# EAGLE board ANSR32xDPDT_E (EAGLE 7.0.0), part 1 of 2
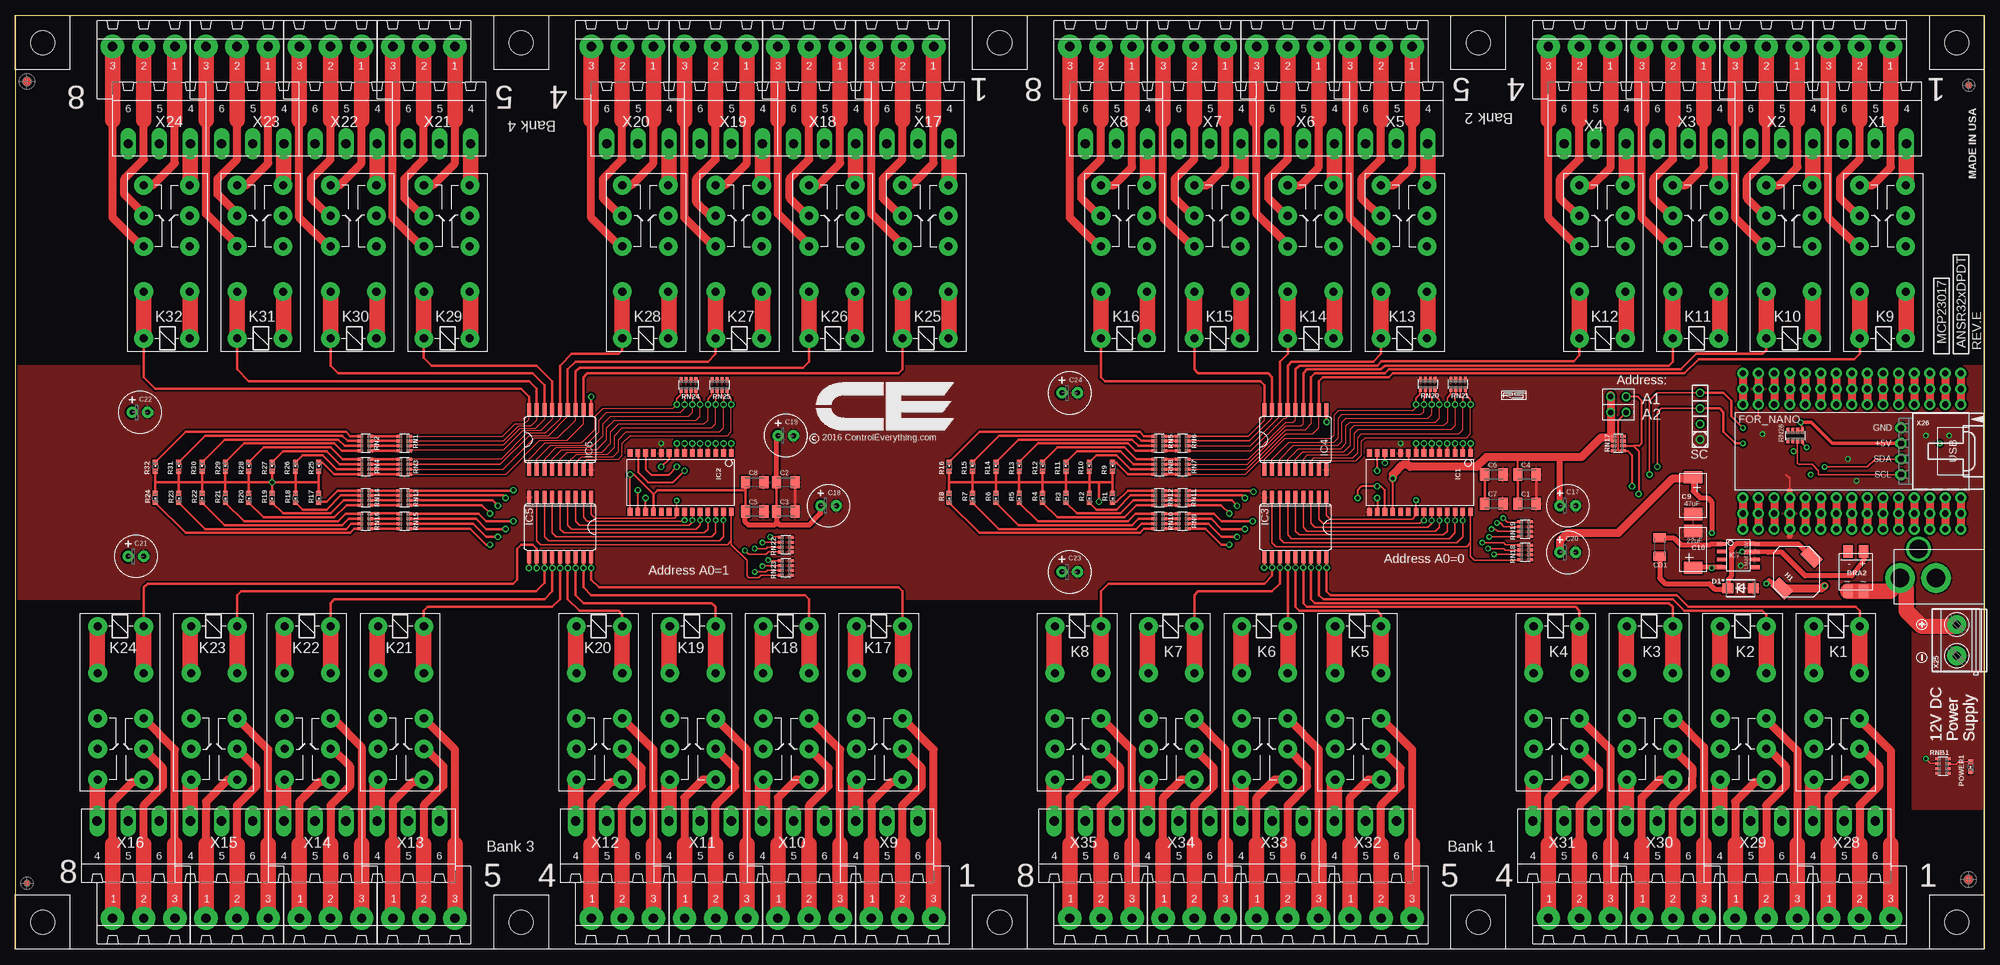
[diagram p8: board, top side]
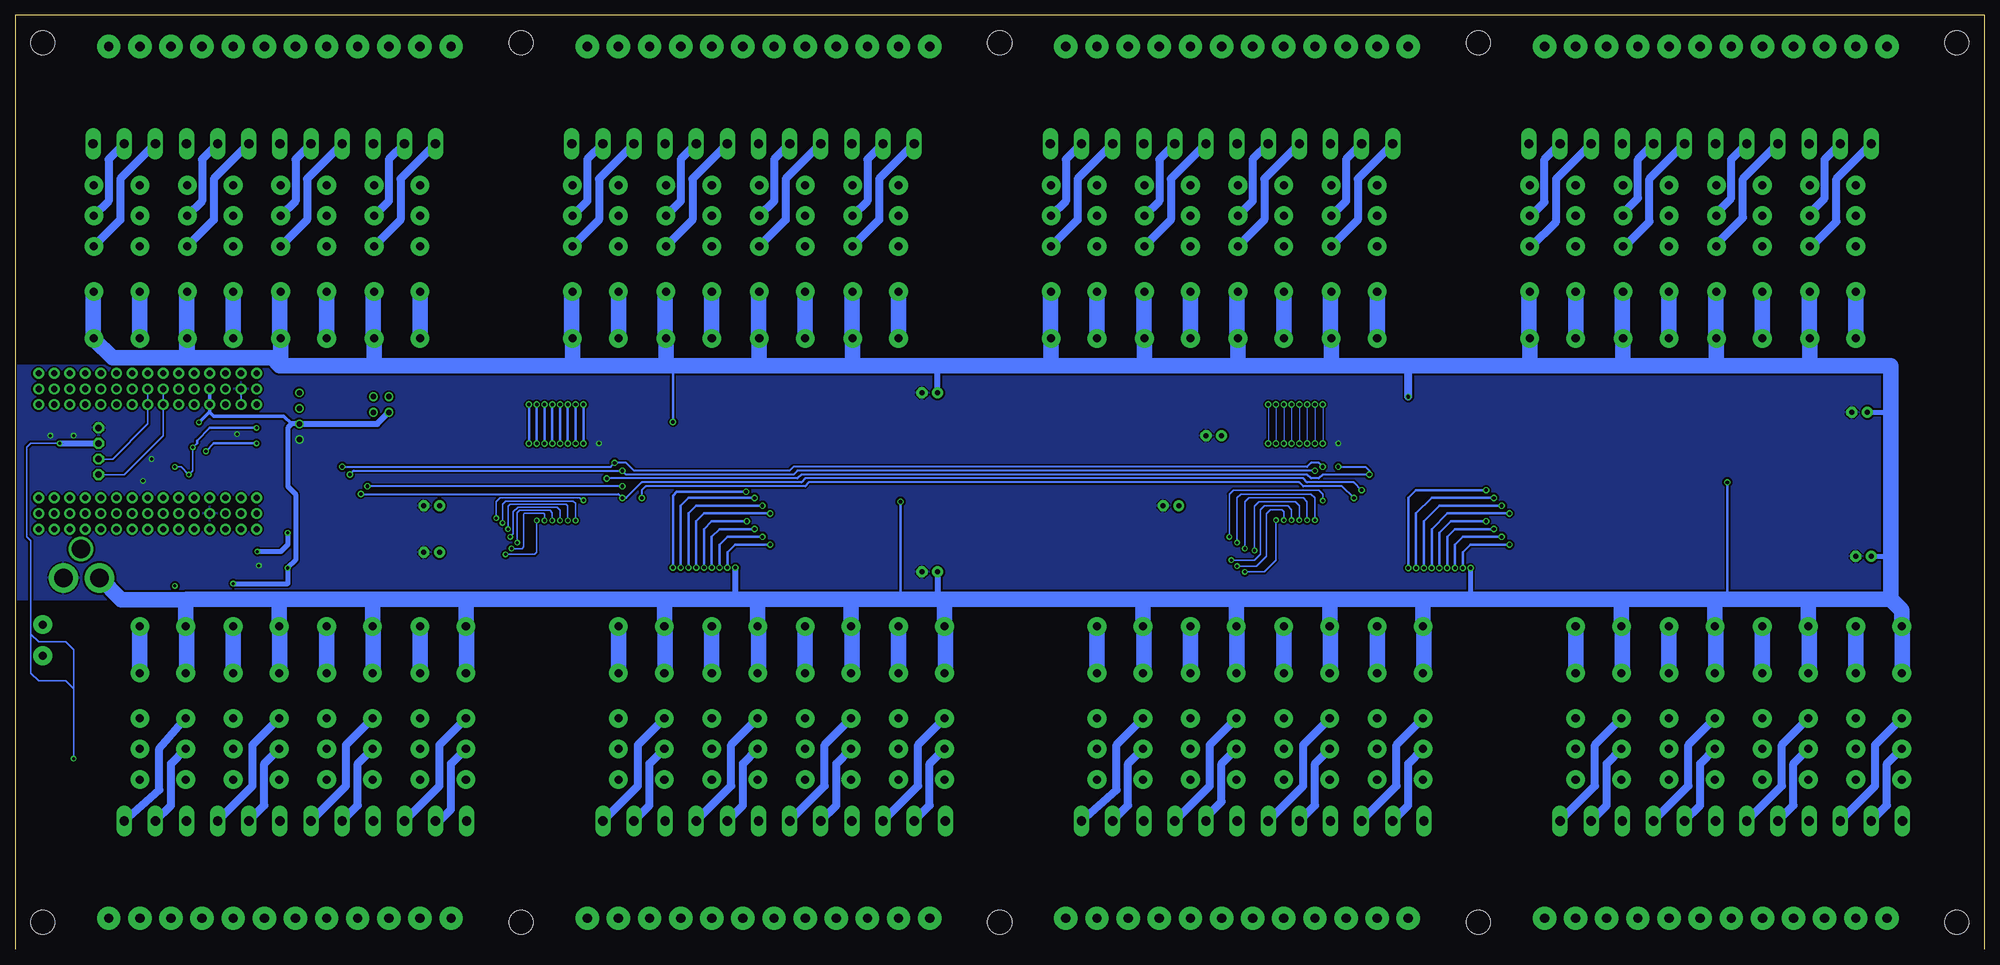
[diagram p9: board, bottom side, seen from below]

Size 321.31 x 152.41 mm. Coordinates in mm from the lower left corner, seen from the top.
Outline: 321.29,0 321.29,152.41 0,152.41 0,0.01
Outline: 321.29,93.99 321.29,13.97
Outline: 321.29,95.26 321.29,14.6
Outline: 321.31,95.26 321.31,37.48
Copper layers (1*16): Top 0.035mm / dielectric 1.5mm / Bottom 0.035mm
Design rules "default": minimum track width 5mil, minimum drill 24mil, track to track 5mil, track to pad 5mil, pad to pad 5mil, via to via 5mil, smd to smd 5mil, copper to edge 10mil, drill to drill 8mil, minimum pad ring 10mil, minimum via ring 8mil, stop-mask expansion 2mil, vias tented up to drill 0mil, thermal gap 10mil

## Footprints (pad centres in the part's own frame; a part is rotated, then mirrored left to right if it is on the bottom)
MB2S = smd 1.55 x 2.1: + 0,-6.5; - 2.54,-6.5; ~@1 0,0; ~@2 2.54,0
_CA_.1UF_50V = smd 1.5 x 2: 1 -1.5,0; 2 1.5,0
_CB_10UF_25V = smd 1.5 x 2: 1 -1.5,0; 2 1.5,0
C2917(7343)-Y = smd 2 x 3: 1 -3,0; 2 3,0
E-025X060 = drill 0.813 pad 1.778: + -1.27,0 | drill 0.813 pad 1.778 octagon: - 1.27,0
_CD_10NF_50V = smd 1.5 x 2: 1 -1.5,0; 2 1.5,0
DO214AC_ZENER = smd 1.8 x 1.7: A 2.05,0; C -2.05,0
ARDUINO_NANO = drill 1 pad 1.778: 3V1 -2.54,-2.54; 3V3 0,-2.54; 5V 0,-27.94; 5V1 -2.54,-27.94; A0 0,-7.62; A1 0,-10.16; A2 0,-12.7; A3 0,-15.24; A4 0,-17.78; A5 0,-20.32; A6 0,-22.86; A7 0,-25.4; A8 -2.54,-7.62; A9 -2.54,-10.16; A10 -2.54,-12.7; A11 -2.54,-15.24; A12 -2.54,-17.78; A13 -2.54,-20.32; A14 -2.54,-22.86; A15 -2.54,-25.4; D1 -2.54,0; D2 20.32,-25.4; D3 20.32,-22.86; D4 20.32,-20.32; D5 20.32,-17.78; D6 20.32,-15.24; D7 20.32,-12.7; D8 20.32,-10.16; D9 20.32,-7.62; D10 20.32,-5.08; D11 20.32,-2.54; D12 20.32,0; D13 0,0; D14 22.86,0; D15 22.86,-2.54; D16 22.86,-5.08; D17 22.86,-7.62; D18 22.86,-10.16; D19 22.86,-12.7; D20 22.86,-15.24; D21 22.86,-17.78; D22 22.86,-20.32; D23 22.86,-22.86; D24 22.86,-25.4; GND 0,-33.02; GND1 -2.54,-33.02; GND@1 20.32,-27.94; GND@2 22.86,-27.94; P$16 2.54,0; P$17 2.54,-2.54; P$18 2.54,-5.08; P$19 2.54,-7.62; P$20 2.54,-10.16; P$21 2.54,-12.7; P$22 2.54,-15.24; P$23 2.54,-17.78; P$24 2.54,-20.32; P$25 2.54,-22.86; P$26 2.54,-25.4; P$27 2.54,-27.94; P$28 2.54,-30.48; P$29 2.54,-33.02; P$30 2.54,-35.56; P$31 17.78,0; P$32 17.78,-2.54; P$33 17.78,-5.08; P$34 17.78,-7.62; P$35 17.78,-10.16; P$36 17.78,-12.7; P$37 17.78,-15.24; P$38 17.78,-17.78; P$39 17.78,-20.32; P$40 17.78,-22.86; P$41 17.78,-25.4; P$42 17.78,-27.94; P$43 17.78,-30.48; P$44 17.78,-33.02; P$45 17.78,-35.56; REF 0,-5.08; REF1 -2.54,-5.08; RST 0,-30.48; RST1 -2.54,-30.48; RST@1 20.32,-30.48; RST@2 22.86,-30.48; RX0 20.32,-33.02; RX1 22.86,-33.02; TX1 20.32,-35.56; TX2 22.86,-35.56; VIN 0,-35.56; VIN1 -2.54,-35.56
IND_ELL8TP = smd 2.054 x 3.2 rotated 45: 1 -2.442,-2.696; 2 2.442,2.442
SO28W = smd 0.762 x 1.27: 1 -7.62,-4.78; 2 -6.35,-4.78; 3 -5.08,-4.78; 4 -3.81,-4.78; 5 -2.54,-4.78; 6 -1.27,-4.78; 7 0,-4.78; 8 1.27,-4.78; 9 2.54,-4.78; 10 3.81,-4.78; 11 5.08,-4.78; 12 6.35,-4.78; 13 7.62,-4.78; 14 8.89,-4.78; 15 8.89,4.78; 16 7.62,4.78; 17 6.35,4.78; 18 5.08,4.78; 19 3.81,4.78; 20 2.54,4.78; 21 1.27,4.78; 22 0,4.78; 23 -1.27,4.78; 24 -2.54,4.78; 25 -3.81,4.78; 26 -5.08,4.78; 27 -6.35,4.78; 28 -7.62,4.78
SO18L = smd 0.66 x 2.032: 1 -5.08,-4.902; 2 -3.81,-4.902; 3 -2.54,-4.902; 4 -1.27,-4.902; 5 0,-4.902; 6 1.27,-4.902; 7 2.54,-4.902; 8 3.81,-4.902; 9 5.08,-4.902; 10 5.08,4.902; 11 3.81,4.902; 12 2.54,4.902; 13 1.27,4.902; 14 0,4.902; 15 -1.27,4.902; 16 -2.54,4.902; 17 -3.81,4.902; 18 -5.08,4.902
SO-8 = smd 0.6 x 1.55: 1 -1.905,-2.69; 2 -0.635,-2.69; 3 0.635,-2.69; 4 1.905,-2.69; 5 1.905,2.71; 6 0.635,2.71; 7 -0.635,2.71; 8 -1.905,2.71
G2R2 = drill 1.321 pad 3.048: 1 -2.54,-3.683; 2 -2.54,3.81; 3 5.08,-3.683; 4 5.08,3.81; O1 12.471,3.81; O2 12.471,-3.683; P1 17.45,3.81; P2 17.45,-3.683; S1 22.454,3.81; S2 22.454,-3.683
CHIPLED_0603 = smd 0.8 x 0.8: A 0,-0.75; C 0,0.75
RNB = smd 0.5 x 0.9: 1 -1.2,-0.8; 2 -0.4,-0.8; 3 0.4,-0.8; 4 1.2,-0.8; 5 1.2,0.8; 6 0.4,0.8; 7 -0.4,0.8; 8 -1.2,0.8
RNE = smd 0.5 x 0.9: 1 -1.2,-0.8; 2 -0.4,-0.8; 3 0.4,-0.8; 4 1.2,-0.8; 5 1.2,0.8; 6 0.4,0.8; 7 -0.4,0.8; 8 -1.2,0.8
RND = smd 0.5 x 0.9: 1 -1.2,-0.8; 2 -0.4,-0.8; 3 0.4,-0.8; 4 1.2,-0.8; 5 1.2,0.8; 6 0.4,0.8; 7 -0.4,0.8; 8 -1.2,0.8
PCB_MOUNTING_HOLE = hole 3.962: 4.445,4.445
PJ-102A = drill 3 pad 4.8: RING 0.1,-3.39; TIP 0.1,-9.29 | drill 3 pad 3.251: RING_SW -4.6,-6.29
JUMPER_2X2 = drill 0.9: A1 0,2.54; A2 0,0; B1 2.54,2.54; B2 2.54,0
MDSTB3 = drill 1.524 pad 3.81: 1 -3.81,-10.795; 2 1.27,-10.795; 3 6.35,-10.795 | drill 1.524 pad 2.54 long: 4 -6.35,5.08; 5 -1.27,5.08; 6 3.81,5.08
MKDSN1,5/2-5,08 = drill 1.3 pad 3.048: 1 -2.561,0.025; 2 2.519,0.025
70553-04 = drill 1.1 pad 1.778 octagon: 1 -3.81,-7.62; 2 -1.27,-7.62; 3 1.27,-7.62; 4 3.81,-7.62

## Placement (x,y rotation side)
BRA2  MB2S_  [MB2S]  301.62,58.43 180 top
C1  [_CA_.1UF_50V]  246.7,72.72 0 top
C2  _CB_10UF_25VC1206K  [_CB_10UF_25V]  125.73,76.21 0 top
C3  [_CA_.1UF_50V]  125.73,71.45 0 top
C4  _CB_10UF_25VC1206K  [_CB_10UF_25V]  246.7,77.48 0 top
C5  [_CA_.1UF_50V]  120.65,71.45 0 top
C6  _CB_10UF_25VC1206K  [_CB_10UF_25V]  241.3,77.48 0 top
C7  [_CA_.1UF_50V]  241.3,72.72 0 top
C8  _CB_10UF_25VC1206K  [_CB_10UF_25V]  120.65,76.21 0 top
C9  47uF  [C2917(7343)-Y]  273.81,74.05 270 top
C10  22uF  [C2917(7343)-Y]  273.81,65.27 90 top
C17  100uF  [E-025X060]  253.37,72.4 0 top
C18  100uF  [E-025X060]  132.72,72.4 0 top
C19  100uF  [E-025X060]  125.73,83.83 0 top
C20  100uF  [E-025X060]  253.37,64.78 0 top
C21  100uF  [E-025X060]  19.68,64.15 0 top
C22  100uF  [E-025X060]  20.32,87.64 0 top
C23  100uF  [E-025X060]  172.09,61.61 0 top
C24  100uF  [E-025X060]  172.09,90.82 0 top
CD1  [_CD_10NF_50V]  268.35,65.67 270 top
D1  B360A  [DO214AC_ZENER]  281.56,58.94 0 top
FOR_NANO  ARDUINO_NANO  [ARDUINO_NANO]  317.5,91.45 270 top
H1  ELL8TP  [IND_ELL8TP]  290.7,61.61 0 top
IC1  MCP23017SO  [SO28W]  229.87,76.21 180 top
IC2  MCP23017SO  [SO28W]  109.22,76.21 180 top
IC3  ULN2803  [SO18L]  208.91,68.91 180 top
IC4  ULN2803  [SO18L]  208.91,83.2 0 top
IC5  ULN2803  [SO18L]  88.9,68.91 180 top
IC6  ULN2803  [SO18L]  88.9,83.2 0 top
IC7  LM2675-5V  [SO-8]  281.18,64.27 270 top
K1  G2R2  [G2R2]  297.18,50.18 270 top
K2  G2R2  [G2R2]  281.94,50.18 270 top
K3  G2R2  [G2R2]  266.7,50.18 270 top
K4  G2R2  [G2R2]  251.46,50.18 270 top
K5  G2R2  [G2R2]  219.07,50.18 270 top
K6  G2R2  [G2R2]  203.84,50.18 270 top
K7  G2R2  [G2R2]  188.59,50.18 270 top
K8  G2R2  [G2R2]  173.35,50.18 270 top
K9  G2R2  [G2R2]  304.8,102.25 90 top
K10  G2R2  [G2R2]  289.56,102.25 90 top
K11  G2R2  [G2R2]  274.32,102.25 90 top
K12  G2R2  [G2R2]  259.08,102.25 90 top
K13  G2R2  [G2R2]  226.69,102.25 90 top
K14  G2R2  [G2R2]  211.46,102.25 90 top
K15  G2R2  [G2R2]  196.22,102.25 90 top
K16  G2R2  [G2R2]  180.97,102.25 90 top
K17  G2R2  [G2R2]  140.97,50.18 270 top
K18  G2R2  [G2R2]  125.73,50.18 270 top
K19  G2R2  [G2R2]  110.49,50.18 270 top
K20  G2R2  [G2R2]  95.25,50.18 270 top
K21  G2R2  [G2R2]  62.87,50.18 270 top
K22  G2R2  [G2R2]  47.62,50.18 270 top
K23  G2R2  [G2R2]  32.38,50.18 270 top
K24  G2R2  [G2R2]  17.14,50.18 270 top
K25  G2R2  [G2R2]  148.59,102.25 90 top
K26  G2R2  [G2R2]  133.35,102.25 90 top
K27  G2R2  [G2R2]  118.11,102.25 90 top
K28  G2R2  [G2R2]  102.87,102.25 90 top
K29  G2R2  [G2R2]  70.48,102.25 90 top
K30  G2R2  [G2R2]  55.24,102.25 90 top
K31  G2R2  [G2R2]  40.01,102.25 90 top
K32  G2R2  [G2R2]  24.77,102.25 90 top
POWER1  LED_NCD  [CHIPLED_0603]  319.09,29.86 180 top
R1  LED_NCD  [CHIPLED_0603]  179.07,73.67 180 top
R2  LED_NCD  [CHIPLED_0603]  175.26,73.67 180 top
R3  LED_NCD  [CHIPLED_0603]  171.45,73.67 180 top
R4  LED_NCD  [CHIPLED_0603]  167.64,73.67 180 top
R5  LED_NCD  [CHIPLED_0603]  163.83,73.67 180 top
R6  LED_NCD  [CHIPLED_0603]  160.02,73.67 180 top
R7  LED_NCD  [CHIPLED_0603]  156.21,73.67 180 top
R8  LED_NCD  [CHIPLED_0603]  152.4,73.67 180 top
R9  LED_NCD  [CHIPLED_0603]  179.07,78.75 0 top
R10  LED_NCD  [CHIPLED_0603]  175.26,78.75 0 top
R11  LED_NCD  [CHIPLED_0603]  171.45,78.75 0 top
R12  LED_NCD  [CHIPLED_0603]  167.64,78.75 0 top
R13  LED_NCD  [CHIPLED_0603]  163.83,78.75 0 top
R14  LED_NCD  [CHIPLED_0603]  160.02,78.75 0 top
R15  LED_NCD  [CHIPLED_0603]  156.21,78.75 0 top
R16  LED_NCD  [CHIPLED_0603]  152.4,78.75 0 top
R17  LED_NCD  [CHIPLED_0603]  49.53,73.67 180 top
R18  LED_NCD  [CHIPLED_0603]  45.72,73.67 180 top
R19  LED_NCD  [CHIPLED_0603]  41.91,73.67 180 top
R20  LED_NCD  [CHIPLED_0603]  38.1,73.67 180 top
R21  LED_NCD  [CHIPLED_0603]  34.29,73.67 180 top
R22  LED_NCD  [CHIPLED_0603]  30.48,73.67 180 top
R23  LED_NCD  [CHIPLED_0603]  26.67,73.67 180 top
R24  LED_NCD  [CHIPLED_0603]  22.86,73.67 180 top
R25  LED_NCD  [CHIPLED_0603]  49.53,78.75 0 top
R26  LED_NCD  [CHIPLED_0603]  45.72,78.75 0 top
R27  LED_NCD  [CHIPLED_0603]  41.91,78.75 0 top
R28  LED_NCD  [CHIPLED_0603]  38.1,78.75 0 top
R29  LED_NCD  [CHIPLED_0603]  34.29,78.75 0 top
R30  LED_NCD  [CHIPLED_0603]  30.48,78.75 0 top
R31  LED_NCD  [CHIPLED_0603]  26.67,78.75 0 top
R32  LED_NCD  [CHIPLED_0603]  22.86,78.75 0 top
RN1  _RNB_510  [RNB]  63.5,82.56 90 top
RN2  _RNB_510  [RNB]  57.15,82.56 90 top
RN3  _RNB_510  [RNB]  63.5,78.75 270 top
RN4  _RNB_510  [RNB]  57.15,78.75 270 top
RN5  _RNB_510  [RNB]  186.69,82.56 270 top
RN6  _RNB_510  [RNB]  190.5,82.56 270 top
RN7  _RNB_510  [RNB]  190.5,78.75 270 top
RN8  _RNB_510  [RNB]  186.69,78.75 270 top
RN9  _RNB_510  [RNB]  190.5,69.86 270 top
RN10  _RNB_510  [RNB]  186.69,69.86 270 top
RN11  _RNB_510  [RNB]  190.5,73.67 90 top
RN12  _RNB_510  [RNB]  186.69,73.67 90 top
RN13  _RNB_510  [RNB]  63.5,73.67 270 top
RN14  _RNB_510  [RNB]  57.15,73.67 270 top
RN15  _RNB_510  [RNB]  63.5,69.86 270 top
RN16  _RNB_510  [RNB]  57.15,69.86 270 top
RN17  _RNE_10K  [RNE]  261.62,82.56 270 top
RN18  _RNE_10K  [RNE]  246.38,64.78 90 top
RN19  _RNE_10K  [RNE]  246.38,68.59 90 top
RN20  _RNE_10K  [RNE]  230.5,92.21 180 top
RN21  _RNE_10K  [RNE]  235.46,92.21 180 top
RN22  _RNE_10K  [RNE]  125.73,66.05 90 top
RN23  _RNE_10K  [RNE]  125.73,62.24 90 top
RN24  _RNE_10K  [RNE]  109.86,92.09 180 top
RN25  _RNE_10K  [RNE]  114.94,92.09 180 top
RN26  _RND_4.7K  [RND]  290.45,83.83 0 top
RNB1  _RNB_510  [RNB]  314.58,29.92 90 top
U$1  PCB_MOUNTING_HOLE  [PCB_MOUNTING_HOLE]  243.21,143.52 90 top
U$2  2.1MMJACK  [PJ-102A]  316.87,60.72 270 top
U$4  PCB_MOUNTING_HOLE  [PCB_MOUNTING_HOLE]  78.11,8.9 270 top
U$5  PCB_MOUNTING_HOLE  [PCB_MOUNTING_HOLE]  321.31,143.52 90 top
U$6  PCB_MOUNTING_HOLE  [PCB_MOUNTING_HOLE]  0,8.9 270 top
U$7  PCB_MOUNTING_HOLE  [PCB_MOUNTING_HOLE]  87,143.52 90 top
U$8  PCB_MOUNTING_HOLE  [PCB_MOUNTING_HOLE]  8.89,143.52 90 top
U$9  PCB_MOUNTING_HOLE  [PCB_MOUNTING_HOLE]  165.1,143.52 90 top
U$10  PCB_MOUNTING_HOLE  [PCB_MOUNTING_HOLE]  234.31,8.9 270 top
U$11  PCB_MOUNTING_HOLE  [PCB_MOUNTING_HOLE]  312.42,8.9 270 top
U$12  PCB_MOUNTING_HOLE  [PCB_MOUNTING_HOLE]  156.21,8.9 270 top
U$13  JUMPER_2X2  [JUMPER_2X2]  260.35,90.18 270 top
U$15  [VISION_REF15]  318.77,11.44 90 top
U$17  [ICON_MINUS]  311.15,47.64 90 top
U$18  [VISION_REF10]  318.77,140.98 90 top
U$19  [ICON_PLUS]  311.15,53.04 0 top
U$21  [ICON_USA]  320.04,125.74 90 top
U$22  [ICON_MINUS]  311.15,47.64 90 top
U$23  [VISION_REF15]  1.91,141.62 90 top
U$24  [ICON_PLUS]  311.15,53.04 0 top
U$25  [ICON_MINUS]  311.15,47.64 90 top
U$26  [ICON_PLUS]  311.15,53.04 0 top
U$28  [VISION_REF10]  1.91,10.81 90 top
X1  MDSTB3  [MDSTB3]  302.26,136.54 180 top
X2  MDSTB3  [MDSTB3]  287.02,136.54 180 top
X3  MDSTB3  [MDSTB3]  271.78,136.54 180 top
X4  MDSTB3  [MDSTB3]  256.54,136.54 180 top
X5  MDSTB3  [MDSTB3]  224.16,136.54 180 top
X6  MDSTB3  [MDSTB3]  208.91,136.54 180 top
X7  MDSTB3  [MDSTB3]  193.68,136.54 180 top
X8  MDSTB3  [MDSTB3]  178.44,136.54 180 top
X9  MDSTB3  [MDSTB3]  143.51,15.89 0 top
X10  MDSTB3  [MDSTB3]  128.27,15.89 0 top
X11  MDSTB3  [MDSTB3]  113.03,15.89 0 top
X12  MDSTB3  [MDSTB3]  97.79,15.89 0 top
X13  MDSTB3  [MDSTB3]  65.41,15.89 0 top
X14  MDSTB3  [MDSTB3]  50.16,15.89 0 top
X15  MDSTB3  [MDSTB3]  34.92,15.89 0 top
X16  MDSTB3  [MDSTB3]  19.68,15.89 0 top
X17  MDSTB3  [MDSTB3]  146.05,136.54 180 top
X18  MDSTB3  [MDSTB3]  130.81,136.54 180 top
X19  MDSTB3  [MDSTB3]  115.57,136.54 180 top
X20  MDSTB3  [MDSTB3]  100.33,136.54 180 top
X21  MDSTB3  [MDSTB3]  67.94,136.54 180 top
X22  MDSTB3  [MDSTB3]  52.7,136.54 180 top
X23  MDSTB3  [MDSTB3]  37.47,136.54 180 top
X24  MDSTB3  [MDSTB3]  22.23,136.54 180 top
X25  MKDSN1,5/2-5,08  [MKDSN1,5/2-5,08]  316.87,50.5 90 top
X26  C-GRID-04-70553  [70553-04]  315.34,81.29 270 top
X28  MDSTB3  [MDSTB3]  299.72,15.89 0 top
X29  MDSTB3  [MDSTB3]  284.48,15.89 0 top
X30  MDSTB3  [MDSTB3]  269.24,15.89 0 top
X31  MDSTB3  [MDSTB3]  254,15.89 0 top
X32  MDSTB3  [MDSTB3]  221.62,15.89 0 top
X33  MDSTB3  [MDSTB3]  206.38,15.89 0 top
X34  MDSTB3  [MDSTB3]  191.13,15.89 0 top
X35  MDSTB3  [MDSTB3]  175.9,15.89 0 top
